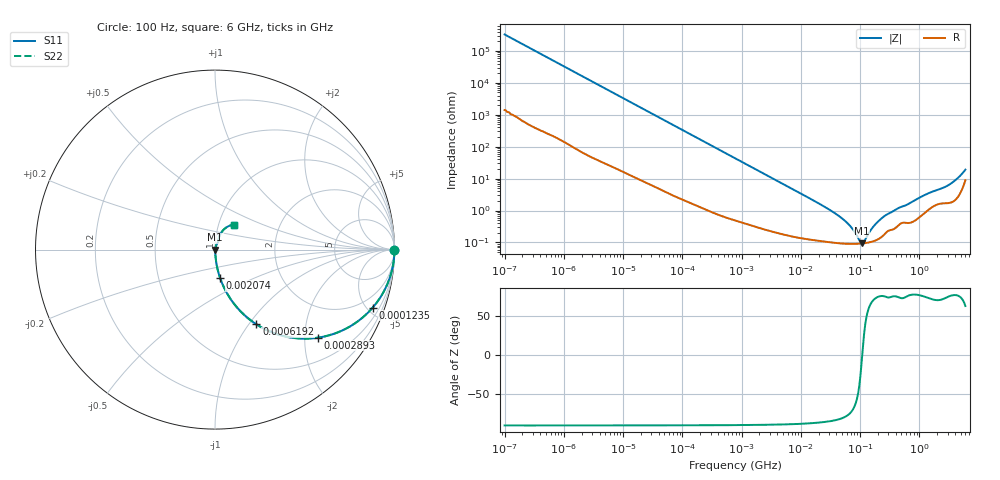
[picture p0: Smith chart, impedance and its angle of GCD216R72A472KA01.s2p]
!Murata Part Number: GCD216R72A472KA01
!These Parameters are Measured in Series Mode Connection
!Data Generated on Mar 13, 2026
!  o--ll--o
!Port1  Port2
!  o------o
!Operation Temp=25[degC], DC Bias Voltage=0[V]
!Freq. Start=100[Hz] Stop=6[GHz] 401[Steps]
# Hz S RI R 50
!Freq.(Hz) S11(Real) S11(Imag) S21(Real) S21(Imag) S12(Real) S12(Imag) S22(Real) S22(Imag)
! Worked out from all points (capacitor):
!   401 points, 100 Hz to 6 GHz, reference 50 ohm
!   read as one part in series: C = 4.85 nF near 109 Hz
!   lowest |Z| = 93.8 mohm at 106.7 MHz (marker M1)
!   series resonance near 108.9 MHz, so ESL is about 440 pH
!   S11 on the Smith chart (normalised r, x): 100 Hz: open; 123.5 kHz: 1.04, -5.41; 289.3 kHz: 1.02, -2.32; 619.2 kHz: 1.01, -1.09; 2.074 MHz: 1.01, -0.33; 6 GHz: 1.18, +0.34
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100  1 -0.000305  1.4e-06 0.000305  1.4e-06 0.000305  1 -0.000305
2008  0.9999 -0.00608  6.18e-05 0.00608  6.18e-05 0.00608  0.9999 -0.00608
12592  0.9984 -0.0379  0.00163 0.0379  0.00163 0.0379  0.9984 -0.0379
40335  0.9849 -0.1192  0.0151 0.1192  0.0151 0.1192  0.9849 -0.1192
123542  0.8782 -0.3236  0.1218 0.3236  0.1218 0.3236  0.8782 -0.3236
289253  0.5733 -0.4905  0.4267 0.4905  0.4267 0.4905  0.5733 -0.4905
619225  0.2306 -0.4161  0.7694 0.4161  0.7694 0.4161  0.2306 -0.4161
774597  0.1621 -0.363  0.8379 0.363  0.8379 0.363  0.1621 -0.363
2074311  0.0286 -0.1585  0.9714 0.1585  0.9714 0.1585  0.0286 -0.1585
1.555665e7  0.00167 -0.0217  0.9983 0.0217  0.9983 0.0217  0.00167 -0.0217
3.330331e7  0.00109 -0.00951  0.9989 0.00951  0.9989 0.00951  0.00109 -0.00951
5.449875e7  0.00094 -0.00484  0.9991 0.00484  0.9991 0.00484  0.00094 -0.00484
7.129496e7  0.000909 -0.00283  0.9991 0.00283  0.9991 0.00283  0.000909 -0.00283
9.753859e7  0.000916 -0.000716  0.9991 0.000716  0.9991 0.000716  0.000916 -0.000716
1.066761e8  0.000928 -0.000131  0.9991 0.000131  0.9991 0.000131  0.000928 -0.000131
1.166697e8  0.000945 0.000454  0.9991 -0.000454  0.9991 -0.000454  0.000945 0.000454
1.526266e8  0.00104 0.00226  0.999 -0.00226  0.999 -0.00226  0.00104 0.00226
1.909225e8  0.00121 0.00392  0.9988 -0.00392  0.9988 -0.00392  0.00121 0.00392
3.124326e8  0.00246 0.00785  0.9975 -0.00785  0.9975 -0.00785  0.00246 0.00785
1.251881e9  0.00943 0.0294  0.9906 -0.0294  0.9906 -0.0294  0.00943 0.0294
2.931063e9  0.0197 0.0544  0.9803 -0.0544  0.9803 -0.0544  0.0197 0.0544
6e9  0.1032 0.139  0.8968 -0.139  0.8968 -0.139  0.1032 0.139
